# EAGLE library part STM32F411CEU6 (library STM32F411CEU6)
32-Bit MCU 512K Flash 100MHz UFQFPN48 STMicroelectronics STM32F411CEU6, 32bit ARM Cortex M4 MCU, 100MHz, 512 kB Flash, 48-Pin UFQFPN Source: Datasheet
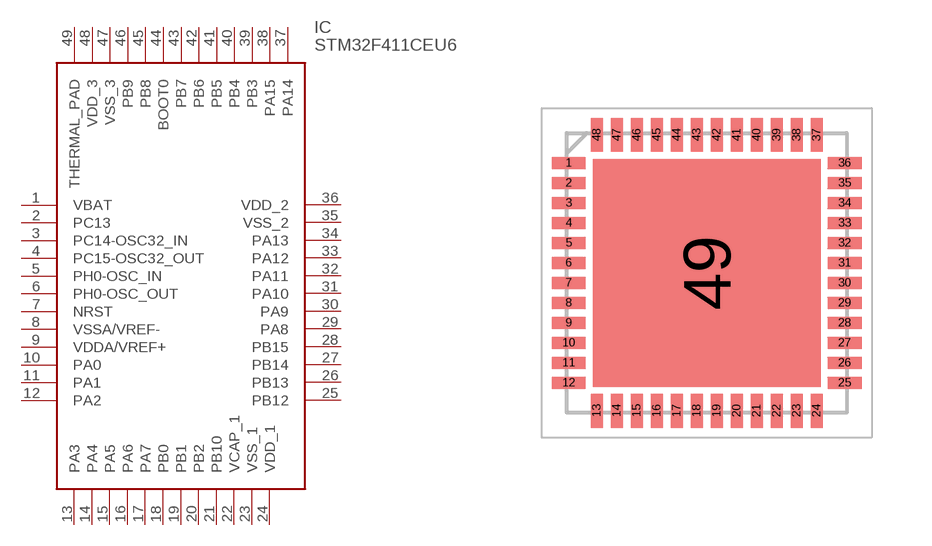
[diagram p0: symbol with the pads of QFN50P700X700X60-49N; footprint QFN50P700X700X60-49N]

Designator prefix IC

## STM32F411CEU6 (Arrow_Part_Number: STM32F411CEU6; Arrow_Price-Stock: https://www.arrow.com/en/products/stm32f411ceu6/stmicroelectronics?utm_currency=USD&region=nac; Description: 32-Bit MCU 512K Flash 100MHz UFQFPN48 STMicroelectronics STM32F411CEU6, 32bit ARM Cortex M4 MCU, 100MHz, 512 kB Flash, 48-Pin UFQFPN; Height: 0.6mm; Manufacturer_Name: STMicroelectronics; Manufacturer_Part_Number: STM32F411CEU6; Mouser_Part_Number: 511-STM32F411CEU6; Mouser_Price-Stock: https://www.mouser.co.uk/ProductDetail/STMicroelectronics/STM32F411CEU6?qs=pjMTYa9MTGV3ou31YBFa3g%3D%3D)  [QFN50P700X700X60-49N]
1  VBAT
2  PC13
3  PC14-OSC32_IN
4  PC15-OSC32_OUT
5  PH0-OSC_IN
6  PH0-OSC_OUT
7  NRST
8  VSSA/VREF-
9  VDDA/VREF+
10  PA0
11  PA1
12  PA2
13  PA3
14  PA4
15  PA5
16  PA6
17  PA7
18  PB0
19  PB1
20  PB2
21  PB10
22  VCAP_1
23  VSS_1
24  VDD_1
25  PB12
26  PB13
27  PB14
28  PB15
29  PA8
30  PA9
31  PA10
32  PA11
33  PA12
34  PA13
35  VSS_2
36  VDD_2
37  PA14
38  PA15
39  PB3
40  PB4
41  PB5
42  PB6
43  PB7
44  BOOT0
45  PB8
46  PB9
47  VSS_3
48  VDD_3
49  THERMAL_PAD

## Footprint QFN50P700X700X60-49N (pad centres in mm)
UFQFPN48_1
smd 0.85 x 0.3: 1 -3.45,2.75; 2 -3.45,2.25; 3 -3.45,1.75; 4 -3.45,1.25; 5 -3.45,0.75; 6 -3.45,0.25; 7 -3.45,-0.25; 8 -3.45,-0.75; 9 -3.45,-1.25; 10 -3.45,-1.75; 11 -3.45,-2.25; 12 -3.45,-2.75; 25 3.45,-2.75; 26 3.45,-2.25; 27 3.45,-1.75; 28 3.45,-1.25; 29 3.45,-0.75; 30 3.45,-0.25; 31 3.45,0.25; 32 3.45,0.75; 33 3.45,1.25; 34 3.45,1.75; 35 3.45,2.25; 36 3.45,2.75
smd 0.3 x 0.85: 13 -2.75,-3.45; 14 -2.25,-3.45; 15 -1.75,-3.45; 16 -1.25,-3.45; 17 -0.75,-3.45; 18 -0.25,-3.45; 19 0.25,-3.45; 20 0.75,-3.45; 21 1.25,-3.45; 22 1.75,-3.45; 23 2.25,-3.45; 24 2.75,-3.45; 37 2.75,3.45; 38 2.25,3.45; 39 1.75,3.45; 40 1.25,3.45; 41 0.75,3.45; 42 0.25,3.45; 43 -0.25,3.45; 44 -0.75,3.45; 45 -1.25,3.45; 46 -1.75,3.45; 47 -2.25,3.45; 48 -2.75,3.45
smd 5.7 x 5.7: 49 0,0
